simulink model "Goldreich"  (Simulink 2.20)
settings: Solver=ode45  StartTime=0.0  StopTime=1  MaxStep=.0005  RelTol=1e-6  AbsTol=1e-6
libraries: simulink x5

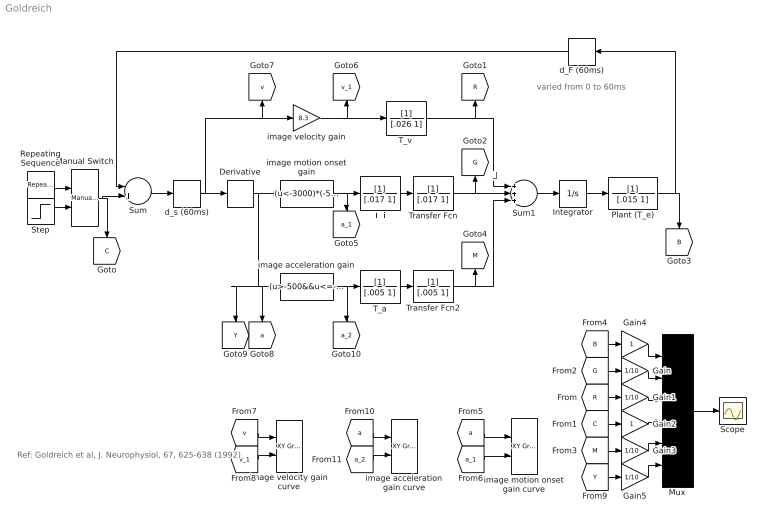
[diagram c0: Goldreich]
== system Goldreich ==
  note: 
  note: Ref: Goldreich et al, J. Neurophysiol, 67, 625-638 (1992)
  note: varied from 0 to 60ms
  Derivative : Derivative
  Gain{,1,3,5} (4 alike) : Gain  Gain=1/10
  Gain2 : Gain  Gain=1
  Gain4 : Gain  Gain=1
  Integrator : Integrator  ExternalReset=none  InitialConditionSource=internal  InitialCondition=0  LimitOutput=off  UpperSaturationLimit=inf  LowerSaturationLimit=-inf  ShowSaturationPort=off  ShowStatePort=off  AbsoluteTolerance=auto
  Manual Switch : simulink/Nonlinear/Manual Switch  sw=1  action=0
  Mux : Mux  Inputs=6
  Plant (T_e) : TransferFcn  Numerator=[1]  Denominator=[.015 1]
  Repeating Sequence : simulink/Sources/Repeating Sequence  rep_seq_t=[0 .1 .10001 2 2.00001 4]  rep_seq_y=[0 0 20 20 0 0]
  Scope : Scope
  Step : Step  Time=1  Before=0  After=1
  Sum : Sum  Inputs=-+
  Sum1 : Sum  Inputs=+++
  T_a : TransferFcn  Numerator=[1]  Denominator=[.005 1]
  T_i : TransferFcn  Numerator=[1]  Denominator=[.017 1]
  "T_v " : TransferFcn  Numerator=[1]  Denominator=[.026 1]
  Transfer Fcn : TransferFcn  Numerator=[1]  Denominator=[.017 1]
  Transfer Fcn2 : TransferFcn  Numerator=[1]  Denominator=[.005 1]
  d_F (60ms) : TransportDelay  Orientation=left  DelayTime=60e-3  InitialInput=0  BufferSize=1024
  d_s (60ms) : TransportDelay  DelayTime=60e-3  InitialInput=0  BufferSize=1024
  image acceleration gain : Fcn  Expr=(u>-500&&u<=-25)*(-42*log(.1*abs(u)+1))+(u>-25&&u<=0)*(-(.0672*u^2)*log(.1*abs(u)+1))+(u>0&&u<=25)*((.0672*u^2)*log(.1*abs(u)+1))+(u>25&&u<=500)*(42*log(.1*abs(u)+1))
  image acceleration gain curve : simulink/Sinks/XY Graph  xmin=-800  xmax=800  ymin=-200  ymax=200  st=.01
  image motion onset gain : Fcn  Expr=(u<-3000)*(-5625*log(.00015*abs(u)+1))+(u>3000)*(5625*log(.00015*abs(u)+1))
  image motion onset gain curve : simulink/Sinks/XY Graph  xmin=-10000  xmax=10000  ymin=-6000  ymax=6000  st=-1
  image velocity gain : Gain  Gain=8.3
  image velocity gain curve : simulink/Sinks/XY Graph  xmin=-25  xmax=25  ymin=-250  ymax=250  st=.01
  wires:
  Sum/1 -> d_s (60ms)/1
  Integrator/1 -> Plant (T_e)/1
  d_s (60ms)/1 -> Derivative/1, image velocity gain/1, [v]
  Sum1/1 -> Integrator/1
  d_F (60ms)/1 -> Sum/1
  Derivative/1 -> image motion onset gain/1, image acceleration gain/1, [a], [Y]
  Manual Switch/1 -> Sum/2, [C]
  T_i/1 -> Transfer Fcn/1
  Plant (T_e)/1 -> d_F (60ms)/1, [B]
  Mux/1 -> Scope/1
  [a] -> image motion onset gain curve/1
  [a_1] -> image motion onset gain curve/2
  [G] -> Gain/1
  [R] -> Gain1/1
  [C] -> Gain2/1
  [M] -> Gain3/1
  [B] -> Gain4/1
  Gain4/1 -> Mux/1
  Gain/1 -> Mux/2
  Gain1/1 -> Mux/3
  Gain2/1 -> Mux/4
  Gain3/1 -> Mux/5
  [Y] -> Gain5/1
  Gain5/1 -> Mux/6
  [a] -> image acceleration gain curve/1
  [a_2] -> image acceleration gain curve/2
  [v] -> image velocity gain curve/1
  [v_1] -> image velocity gain curve/2
  Repeating Sequence/1 -> Manual Switch/1
  Step/1 -> Manual Switch/2
  "T_v "/1 -> Sum1/1, [R]
  image velocity gain/1 -> "T_v "/1, [v_1]
  T_a/1 -> Transfer Fcn2/1
  image acceleration gain/1 -> T_a/1, [a_2]
  image motion onset gain/1 -> T_i/1, [a_1]
  Transfer Fcn/1 -> Sum1/2, [G]
  Transfer Fcn2/1 -> Sum1/3, [M]
